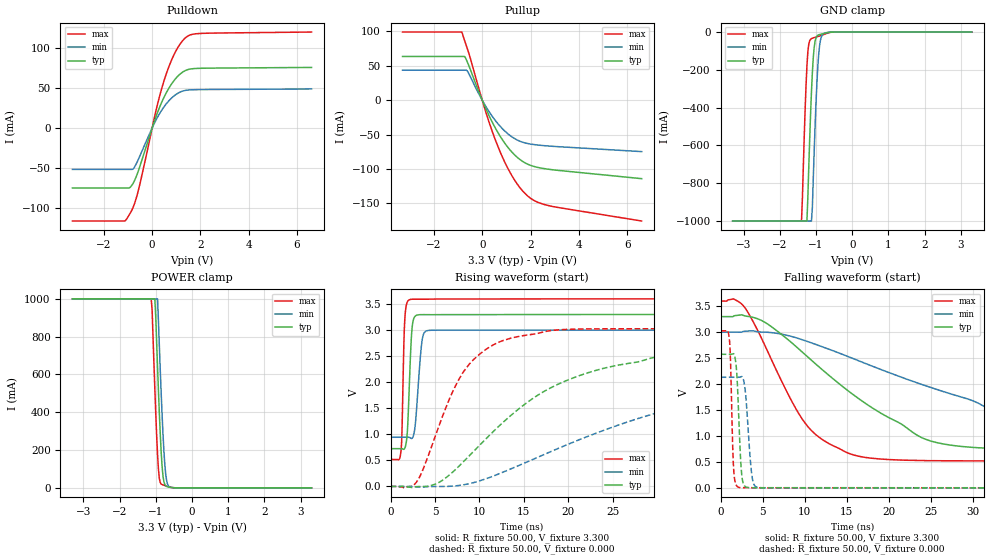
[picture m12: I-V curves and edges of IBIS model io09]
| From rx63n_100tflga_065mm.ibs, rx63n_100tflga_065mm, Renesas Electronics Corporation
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[Model]   io09
Model_type   I/O
Polarity   Non-Inverting
Enable   Active-High
Vinl  =   0.660V
Vinh  =   2.640V
Vmeas =   1.650V
Cref  =   30.00pF
| variable   typ   min   max
C_comp   5.510pF   5.510pF   5.510pF
| variable   typ   min   max
[Temperature Range]   45.000   105.000   -40.000
| variable   typ   min   max
[Voltage Range]   3.300V   3.000V   3.600V
| variable   typ   min   max
[Pullup Reference]   3.300V   3.000V   3.600V
| variable   typ   min   max
[Pulldown Reference]   0.000V   0.000V   0.000V
| variable   typ   min   max
[POWER Clamp Reference] 3.300V   3.000V   3.600V
| variable   typ   min   max
[GND Clamp Reference]   0.000V   0.000V   0.000V
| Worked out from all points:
|   slope of the pulldown table from 0 to 0.495 V, typ, clamps not added: 12.8 ohm
|   slope of the pullup table from 0 to 0.495 V, typ, clamps not added: 13.3 ohm
|   GND clamp passes 1 mA (typ) near -0.60 V on its own axis
|   POWER clamp passes 1 mA (typ) near -0.52 V on its own axis
|   rising waveform, R_fixture 50.00, V_fixture 3.300: 20-80 % time 369ps typ, 539ps min, 248ps max; typ from 0.725 V to 3.3 V
|   rising waveform, R_fixture 50.00, V_fixture 0.000: 20-80 % time 11.8ns typ, 22.7ns min, 4.99ns max; typ from 0 V to 2.57 V
|   falling waveform, R_fixture 50.00, V_fixture 3.300: 20-80 % time 12.8ns typ, 19.7ns min, 6.06ns max; typ from 3.3 V to 0.725 V
|   falling waveform, R_fixture 50.00, V_fixture 0.000: 20-80 % time 415ps typ, 566ps min, 298ps max; typ from 2.57 V to 0 V
[Pulldown]
| io09 Pulldown rx631_rx63n
| Thu Mar 22 17:15:49 2012
| voltage   I(typ)   I(min)   I(max)
-3.3V     -74.79mA   -51.56mA   -116.1mA
-1.125V   -74.79mA   -51.56mA   -116.1mA
-1V       -74.79mA   -51.56mA   -110.9mA
-800mV    -69.71mA   -51.34mA   -99.95mA
-600mV    -55.99mA   -41.07mA   -81.48mA
175mV     15.57mA    10.88mA    23.81mA
525mV     40.57mA    27.99mA    62.24mA
950mV     61.1mA     41.27mA    94.48mA
1.2V      68.64mA    45.61mA    106.9mA
1.4V      72.33mA    47.31mA    113.4mA
2.1V      74.89mA    48.24mA    118.5mA
6.6V      75.9mA     48.99mA    120.2mA
[Pullup]
| io09 Pullup rx631_rx63n
| Thu Mar 22 17:15:49 2012
| voltage   I(typ)   I(min)   I(max)
-3.3V     63.6mA     43.58mA    99.08mA
-850mV    63.6mA     43.58mA    99.08mA
-725mV    63.31mA    43.58mA    86.06mA
-625mV    56.11mA    42.75mA    75.73mA
150mV     -12.34mA   -9.119mA   -17.43mA
650mV     -47.05mA   -34.16mA   -67.27mA
975mV     -64.48mA   -46.14mA   -93.06mA
1.3V      -78.02mA   -54.87mA   -113.9mA
1.925V    -93.62mA   -63.22mA   -140.4mA
2.3V      -97.61mA   -65.11mA   -148.3mA
2.8V      -100.6mA   -66.69mA   -153.5mA
6.6V      -114mA     -74.69mA   -175.5mA
[GND Clamp]
| io09 GNDClamp rx631_rx63n
| Thu Mar 22 17:15:49 2012
| voltage   I(typ)   I(min)   I(max)
-3.3V     -1A        -1A        -1A
-1.4V     -1A        -1A        -1A
-1.3V     -1A        -1A        -412.1mA
-1.25V    -1A        -1A        -179.2mA
-1.2V     -719.8mA   -1A        -65.15mA
-1.15V    -437mA     -1A        -38.52mA
-1.1V     -214.2mA   -928.2mA   -32.63mA
-1.05V    -81.3mA    -631.9mA   -29.36mA
-950mV    -17.38mA   -183.4mA   -23.66mA
-900mV    -13.22mA   -70.92mA   -20.94mA
-825mV    -9.983mA   -15.37mA   -16.48mA
3.3V      0A         0A         0A
[POWER Clamp]
| io09 PWRClamp rx631_rx63n
| Thu Mar 22 17:15:49 2012
| voltage   I(typ)   I(min)   I(max)
-3.3V     1A         1A         1A
-1.125V   1A         1A         1A
-1.1V     1A         1A         941.5mA
-1.025V   1A         1A         524.2mA
-950mV    638.4mA    1A         175.4mA
-900mV    392.9mA    749.3mA    48.84mA
-850mV    189.8mA    501.4mA    20.26mA
-800mV    62.67mA    285.5mA    15.44mA
-750mV    17.75mA    124.3mA    12.1mA
-700mV    7.656mA    38.59mA    8.816mA
-625mV    3.553mA    5.729mA    4.677mA
3.3V      0A         0A         0A
[Ramp]
dV/dt_r   1.544/11.75n   1.278/22.71n   1.815/4.99n
dV/dt_f   1.545/12.85n   1.234/19.69n   1.849/6.05n
R_load = 50.00ohm
[Rising Waveform]
| io09 Rising-High rx631_rx63n
| Thu Mar 22 17:15:49 2012
R_fixture = 50.00
V_fixture = 3.300
V_fixture_min = 3.000
V_fixture_max = 3.600
C_fixture = 0.00pF
| Time   V(typ)   V(min)   V(max)
0s        725mV      944mV      518mV
1.15ns    725mV      944mV      644mV
1.27ns    725mV      944mV      989mV
1.61ns    738mV      944mV      3.229V
1.9ns     1.086V     944mV      3.546V
2.175ns   2.236V     938mV      3.587V
2.6ns     3.217V     992mV      3.593V
3.53ns    3.297V     2.782V     3.594V
4.24ns    3.297V     2.994V     3.594V
80ns      3.3V       3V         3.6V
[Rising Waveform]
| io09 Rising-Low rx631_rx63n
| Thu Mar 22 17:15:49 2012
R_fixture = 50.00
V_fixture = 0.000
C_fixture = 0.00pF
| Time   V(typ)   V(min)   V(max)
0s        0V         0V         0V
3.05ns    -3mV       -8mV       116mV
6.8ns     248mV      4mV        1.748V
8.825ns   583mV      52mV       2.34V
11.41ns   1.03V      190mV      2.704V
14.35ns   1.478V     396mV      2.877V
20.51ns   2.081V     847mV      3.018V
29.87ns   2.485V     1.407V     3.026V
45.32ns   2.573V     2.025V     3.026V
80ns      2.574V     2.131V     3.026V
[Falling Waveform]
| io09 Falling-High rx631_rx63n
| Thu Mar 22 17:15:49 2012
R_fixture = 50.00
V_fixture = 3.300
V_fixture_min = 3.000
V_fixture_max = 3.600
C_fixture = 0.00pF
| Time   V(typ)   V(min)   V(max)
0s        3.3V       3V         3.6V
1.495ns   3.304V     3V         3.642V
2.96ns    3.31V      3.018V     3.453V
5.59ns    3.156V     2.998V     2.627V
8.63ns    2.77V      2.908V     1.616V
10.57ns   2.491V     2.806V     1.142V
16.24ns   1.739V     2.46V      616mV
24.98ns   902mV      1.935V     524mV
39.62ns   733mV      1.08V      519mV
80ns      725mV      944mV      518mV
[Falling Waveform]
| io09 Falling-Low rx631_rx63n
| Thu Mar 22 17:15:49 2012
R_fixture = 50.00
V_fixture = 0.000
C_fixture = 0.00pF
| Time   V(typ)   V(min)   V(max)
0s        2.574V     2.131V     3.026V
1.01ns    2.574V     2.131V     2.894V
1.15ns    2.574V     2.131V     2.527V
1.55ns    2.582V     2.131V     341mV
1.905ns   2.224V     2.13V      37mV
2.2ns     1.147V     2.132V     8mV
2.695ns   80mV       2.092V     3mV
3.715ns   2mV        231mV      3mV
4.52ns    1mV        6mV        1mV
80ns      0V         0V         0V
